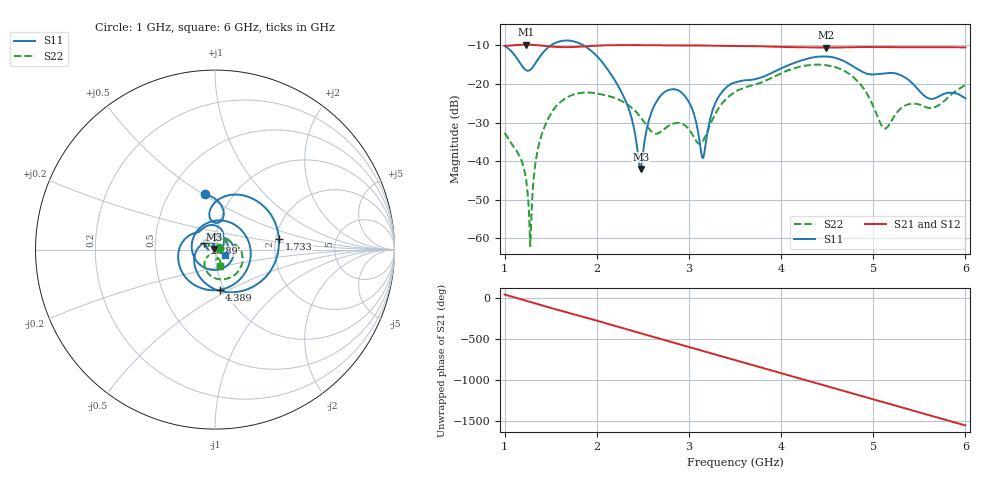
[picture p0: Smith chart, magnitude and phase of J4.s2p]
!Agilent Technologies,E8364B,MY43040528,A.07.50.67
!Agilent E8364B: A.07.50.67
!Date: Sunday, March 01, 2026 19:00:23
!Correction: S11(Full 2 Port(1,2))
!S21(Full 2 Port(1,2))
!S12(Full 2 Port(1,2))
!S22(Full 2 Port(1,2))
!S2P File: Measurements: S11, S21, S12, S22:
# Hz S  dB  R 50
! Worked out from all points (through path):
!   451 points, 1 GHz to 6 GHz, reference 50 ohm
!   highest |S21| = -9.78 dB at 1.233 GHz (marker M1); lowest = -10.5 dB at 4.489 GHz (marker M2)
!   group delay of S21, straight-line fit = 889 ps
!   lowest |S11| = -42.0 dB at 2.478 GHz (marker M3), VSWR 1.02, Z = 49.3 + j0.345 ohm
!   |S11| at or under -10 dB: start of sweep to 1.5 GHz; 1.859 GHz to end of sweep
!   |S22| runs from -62.0 to -14.9 dB; largest |S21 - S12| = 0.0016
!   S11 on the Smith chart (normalised r, x): 1 GHz: 0.74, +0.51; 1.733 GHz: 2.08, +0.30; 2.289 GHz: 0.89, +0.07; 4.389 GHz: 0.95, -0.45; 6 GHz: 1.12, -0.07
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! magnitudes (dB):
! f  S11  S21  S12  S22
! 1 GHz  -10.1  -10.1  -10.2  -32.7
! 1.233 GHz  -16.4  -9.8  -9.8  -44.7
! 1.278 GHz  -16.3  -9.8  -9.8  -62.0
! 1.344 GHz  -14.2  -9.9  -9.9  -39.0
! 1.411 GHz  -12.0  -10.1  -10.1  -32.5
! 1.733 GHz  -8.8  -10.4  -10.4  -22.8
! 1.844 GHz  -9.8  -10.3  -10.3  -22.2
! 2.289 GHz  -23.1  -9.9  -9.9  -24.6
! 2.478 GHz  -42.0  -9.9  -9.9  -28.7
! 2.567 GHz  -29.3  -9.9  -9.9  -31.6
! 2.667 GHz  -23.8  -9.9  -10.0  -32.8
! 2.956 GHz  -23.1  -10.0  -10.0  -30.7
! 3.156 GHz  -39.2  -10.0  -10.0  -34.7
! 3.289 GHz  -24.8  -10.1  -10.1  -27.6
! 3.5 GHz  -19.6  -10.1  -10.2  -22.0
! 4.344 GHz  -13.1  -10.5  -10.5  -15.0
! 4.389 GHz  -12.9  -10.5  -10.5  -14.9
! 4.489 GHz  -12.8  -10.5  -10.6  -15.1
! 4.811 GHz  -15.8  -10.4  -10.5  -18.8
! 5.167 GHz  -17.1  -10.4  -10.5  -30.8
! 5.6 GHz  -23.7  -10.4  -10.5  -26.2
! 6 GHz  -23.7  -10.5  -10.5  -20.2
